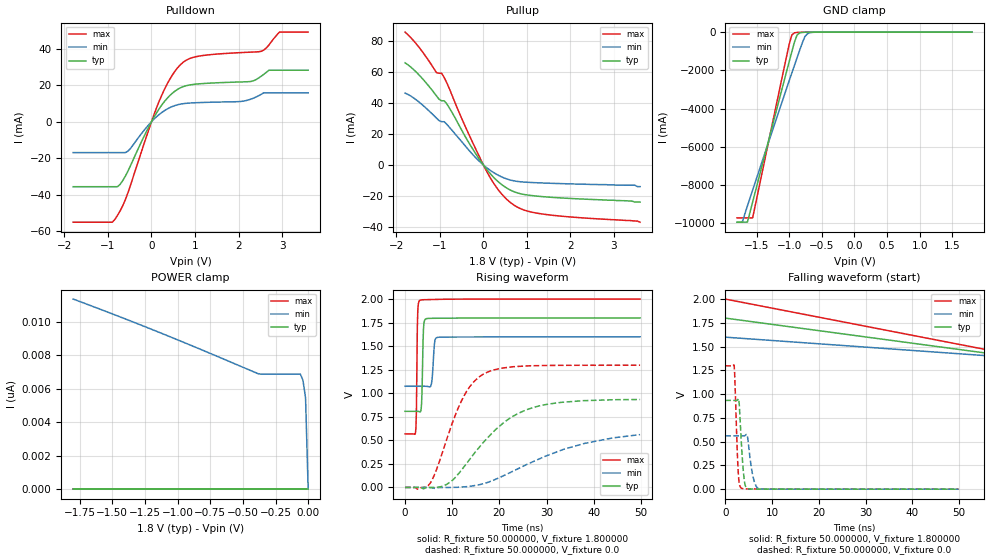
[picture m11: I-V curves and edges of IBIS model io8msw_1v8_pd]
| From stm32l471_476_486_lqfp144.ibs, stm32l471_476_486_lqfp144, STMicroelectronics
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|   Model io8msw_1v8_pd
[Model]  io8msw_1v8_pd
Model_type I/O
Polarity   Non-Inverting
Enable   Active-Low
Vinl =   0.540000V
Vinh =   1.260000V
Vmeas =  0.900000V
Cref =   100.000000nF
Rref =   1.000000k
Vref =   1.800000V
C_comp   2.845500pF   2.787900pF   3.023700pF
[Temperature Range]   25.000000   0.125000k   -40.000000
[Pullup Reference]   1.800000V   1.600000V   2.000000V
[Pulldown Reference]   0.0V   0.0V   0.0V
[POWER Clamp Reference]   1.800000V   1.600000V   2.000000V
[GND Clamp Reference]   0.0V   0.0V   0.0V
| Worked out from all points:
|   slope of the pulldown table from 0 to 0.27 V, typ, clamps not added: 26.4 ohm
|   slope of the pullup table from 0 to 0.27 V, typ, clamps not added: 30.1 ohm
|   GND clamp passes 1 mA (typ) near -0.58 V on its own axis
|   rising waveform, R_fixture 50.000000, V_fixture 1.800000: 20-80 % time 263ps typ, 401ps min, 194ps max; typ from 0.808 V to 1.8 V
|   rising waveform, R_fixture 50.000000, V_fixture 0.0: 20-80 % time 10.6ns typ, 16.4ns min, 6.12ns max; typ from 0 V to 0.933 V
|   falling waveform, R_fixture 50.000000, V_fixture 1.800000: 20-80 % time 90.1ns typ, 90.1ns min, 90.1ns max; typ from 1.8 V to 0.808 V
|   falling waveform, R_fixture 50.000000, V_fixture 0.0: 20-80 % time 712ps typ, 1.02ns min, 552ps max; typ from 0.933 V to 0 V
[Pulldown]
|Voltage   I(typ)   I(min)   I(max)
-1.8V     -35.64mA   -16.93mA   -55.1mA
-840mV    -35.64mA   -16.93mA   -53.52mA
-720mV    -34.31mA   -16.93mA   -48.86mA
-540mV    -27.04mA   -16.13mA   -38.89mA
240mV     9.303mA    5.14mA     14.78mA
480mV     15.67mA    8.374mA    25.64mA
720mV     19.18mA    9.883mA    32.46mA
1.08V     20.76mA    10.49mA    35.95mA
2.1V      21.86mA    11.28mA    37.98mA
2.52V     24.96mA    15.03mA    38.63mA
2.94V     28.26mA    15.88mA    49.18mA
3.6V      28.26mA    15.88mA    49.18mA
[Pullup]
|Voltage   I(typ)   I(min)   I(max)
-1.8V     66.05mA    46.47mA    85.93mA
-1.44V    57.04mA    39.77mA    74.64mA
-1.08V    44.76mA    30.37mA    59.74mA
-960mV    41.53mA    27.97mA    59.32mA
-840mV    39.49mA    26.25mA    53.02mA
-300mV    12.8mA     8.47mA     17.72mA
60mV      -2.268mA   -1.401mA   -3.341mA
300mV     -9.801mA   -6.008mA   -14.46mA
600mV     -15.96mA   -9.582mA   -23.81mA
900mV     -18.89mA   -10.98mA   -28.81mA
1.32V     -20.37mA   -11.6mA    -31.56mA
3.6V      -24mA      -14mA      -37mA
[GND_clamp]
|Voltage   I(typ)   I(min)   I(max)
-1.8V     -9.93A     -9.932A    -9.707A
-1.72V    -9.93A     -9.932A    -9.707A
-1.64V    -9.93A     -9.083A    -9.707A
-1.56V    -8.876A    -8.251A    -9.707A
-1V       -1.54A     -2.541A    -631mA
-960mV    -1.028A    -2.139A    -153.8mA
-920mV    -527mA     -1.74A     -39.13mA
-880mV    -155.7mA   -1.344A    -18.02mA
-840mV    -45.33mA   -953mA     -12.69mA
-760mV    -8.431mA   -235mA     -7.631mA
-680mV    -3.453mA   -33.02mA   -3.876mA
1.8V      47.6uA     51.88uA    39.21uA
[POWER_clamp]
|Voltage   I(typ)   I(min)   I(max)
-1.8V     0A         11.37nA    0A
-1.14V    0A         9.374nA    0A
-380mV    0A         6.895nA    0A
-60mV     0A         6.881nA    0A
-40mV     0A         6.518nA    0A
-20mV     0A         5.452nA    0A
0V        0A         0A         0A
[Ramp]
| variable   typ   min   max
dV/dt_r  0.55940/10.62917n   0.31316/16.48745n   0.77826/6.11293n
dV/dt_f  0.58916/9.85069n   0.28200/14.23375n   0.85860/5.41693n
R_load = 50.000000
[Rising Waveform]
R_fixture= 50.000000
V_fixture= 1.800000
V_fixture_min= 1.600000
V_fixture_max= 2.000000
|time   V(typ)   V(min)   V(max)
0s        807.9mV    1.074V     568mV
2.202ns   808mV      1.074V     575.6mV
2.402ns   808mV      1.074V     802.2mV
2.703ns   807.6mV    1.074V     1.881V
3.203ns   801mV      1.074V     1.988V
3.504ns   891.6mV    1.074V     1.991V
3.904ns   1.681V     1.074V     1.992V
4.404ns   1.789V     1.074V     1.993V
6.907ns   1.796V     1.593V     1.996V
49.85ns   1.799V     1.599V     1.999V
[Rising Waveform]
R_fixture= 50.000000
V_fixture= 0.0
V_fixture_min= 0.0
V_fixture_max= 0.0
|time   V(typ)   V(min)   V(max)
0s        3.019nV    73.58nV    2.158nV
5.405ns   -636.2uV   -1.161mV   50.95mV
8.809ns   32.12mV    -265.8uV   506.5mV
12.11ns   193.9mV    4.727mV    933.4mV
14.41ns   344.3mV    17.24mV    1.112V
16.82ns   490.7mV    42.11mV    1.21V
22.12ns   731.5mV    153.9mV    1.276V
28.13ns   861.2mV    295.2mV    1.293V
38.14ns   921.3mV    468.3mV    1.297V
49.85ns   933.5mV    560.6mV    1.297V
[Falling Waveform]
R_fixture= 50.000000
V_fixture= 1.800000
V_fixture_min= 1.600000
V_fixture_max= 2.000000
|time   V(typ)   V(min)   V(max)
0s        1.799V     1.599V     1.999V
150.2ns   807.9mV    1.074V     568mV
300.3ns   807.9mV    1.074V     568mV
14.86us   807.9mV    1.074V     568mV
[Falling Waveform]
R_fixture= 50.000000
V_fixture= 0.0
V_fixture_min= 0.0
V_fixture_max= 0.0
|time   V(typ)   V(min)   V(max)
0s        933.5mV    560.6mV    1.297V
1.902ns   933.5mV    560.6mV    1.303V
2.803ns   951.7mV    560.6mV    158.6mV
3.003ns   886.7mV    560.6mV    56.81mV
3.504ns   440.2mV    560.4mV    9.543mV
4.304ns   34.8mV     566.5mV    3.16mV
4.705ns   7.8mV      564.9mV    2.703mV
6.106ns   1.014mV    98.84mV    2.221mV
7.207ns   812.4uV    4.249mV    2.119mV
49.85ns   3.019nV    73.58nV    2.158nV
